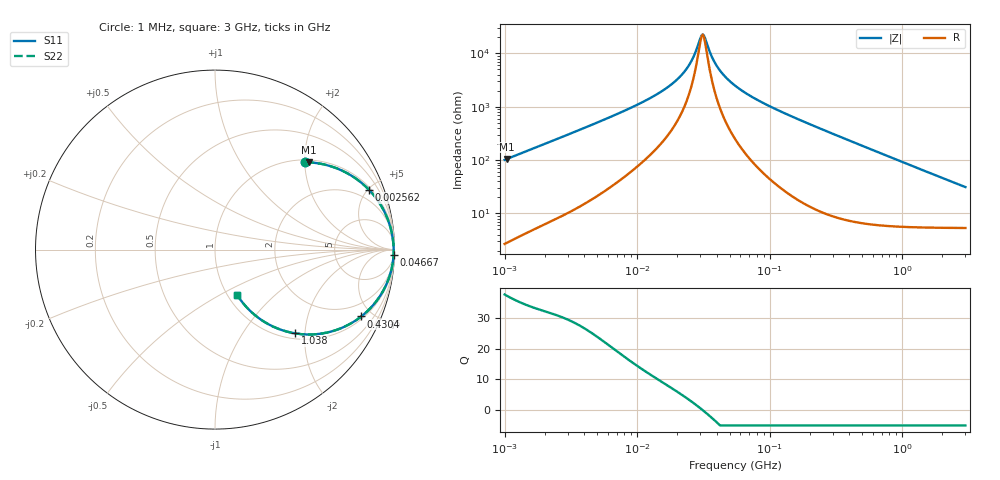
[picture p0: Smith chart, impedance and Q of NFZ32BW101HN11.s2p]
! NFZ32BW101HN11
# Hz S RI R 50
!Freq.(Hz) S11(Real) S11(Imag) S21(Real) S21(Imag) S12(Real) S12(Imag) S22(Real) S22(Imag)
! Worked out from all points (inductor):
!   401 points, 1 MHz to 3 GHz, reference 50 ohm
!   read as one part in series: L = 15.9 uH near 1.041 MHz
!   highest Q = 37.2 at 1.041 MHz (marker M1), where L = 16 uH
!   self-resonance near 30.65 MHz
!   S11 on the Smith chart (normalised r, x): 1 MHz: 1.05, +2.01; 2.562 MHz: 1.17, +5.11; 46.67 MHz: 11, -70; 430.4 MHz: 1.14, -4.30; 1.038 GHz: 1.11, -1.78; 3 GHz: 1.11, -0.61
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1000000  0.5037 0.4869  0.4963 -0.4869  0.4963 -0.4869  0.5037 0.4869
1040844  0.5229 0.4862  0.4771 -0.4862  0.4771 -0.4862  0.5229 0.4862
2561897  0.8594 0.3317  0.1406 -0.3317  0.1406 -0.3317  0.8594 0.3317
3823119  0.9284 0.24  0.0716 -0.24  0.0716 -0.24  0.9284 0.24
8513927  0.9814 0.1083  0.0186 -0.1083  0.0186 -0.1083  0.9814 0.1083
1.461624e7  0.9914 0.0543  0.00858 -0.0543  0.00858 -0.0543  0.9914 0.0543
1.896016e7  0.9937 0.0341  0.00631 -0.0341  0.00631 -0.0341  0.9937 0.0341
2.316168e7  0.9948 0.02  0.00521 -0.02  0.00521 -0.02  0.9948 0.02
2.611722e7  0.9952 0.0119  0.00477 -0.0119  0.00477 -0.0119  0.9952 0.0119
3.00453e7  0.9955 0.00253  0.00446 -0.00253  0.00446 -0.00253  0.9955 0.00253
3.127247e7  0.9956 -0.000123  0.0044 0.000123  0.0044 0.000123  0.9956 -0.000123
3.254976e7  0.9956 -0.00279  0.00436 0.00279  0.00436 0.00279  0.9956 -0.00279
3.897472e7  0.9956 -0.0149  0.00441 0.0149  0.00441 0.0149  0.9956 -0.0149
4.666789e7  0.9952 -0.0276  0.00483 0.0276  0.00483 0.0276  0.9952 -0.0276
5.477226e7  0.9944 -0.0396  0.00558 0.0396  0.00558 0.0396  0.9944 -0.0396
9.034013e7  0.9886 -0.0848  0.0114 0.0848  0.0114 0.0848  0.9886 -0.0848
2.094008e8  0.9476 -0.2091  0.0524 0.2091  0.0524 0.2091  0.9476 -0.2091
4.304467e8  0.8147 -0.3727  0.1853 0.3727  0.1853 0.3727  0.8147 -0.3727
8.005644e8  0.5677 -0.471  0.4323 0.471  0.4323 0.471  0.5677 -0.471
1.038491e9  0.4452 -0.4665  0.5548 0.4665  0.5548 0.4665  0.4452 -0.4665
1.782824e9  0.2351 -0.3751  0.7649 0.3751  0.7649 0.3751  0.2351 -0.3751
3e9  0.125 -0.2551  0.875 0.2551  0.875 0.2551  0.125 -0.2551
